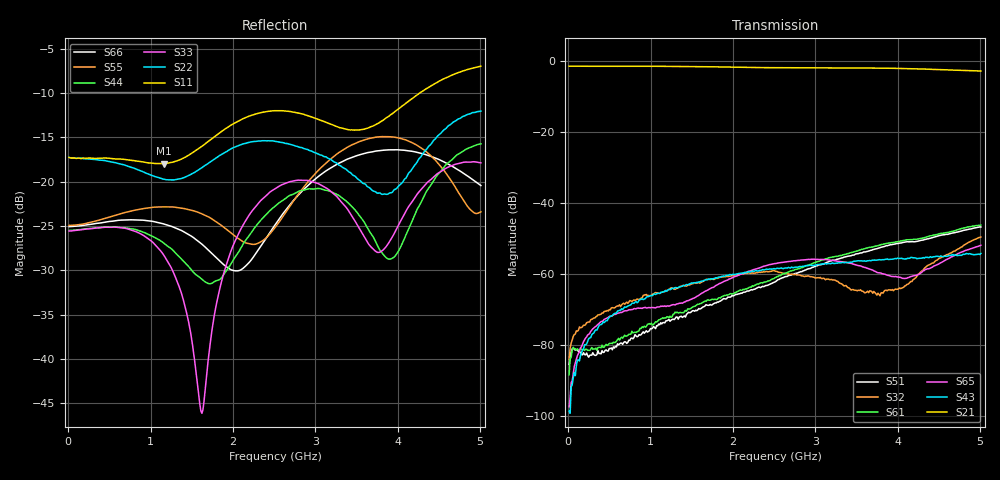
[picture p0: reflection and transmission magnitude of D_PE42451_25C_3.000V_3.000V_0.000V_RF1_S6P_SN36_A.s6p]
! Device ID: PE42451
! Serial: 36
! Insertion: A
! Temp: 25C
! VDD: 3.000
! Control_Hi: 100.000
! Control_Lo: 0.000
! Logic State: RF1
! Port 1: RFC
! Port 2: RF1
! Port 3: RF2
! Port 4: RF3
! Port 5: RF4
! Port 6: RF5
! V1 = 3.00
! V2 = 0.00
! V3 = 0.00
! V4 = 0.00
! IDD: 1.334020e-05
#  Hz  S  RI  R  50
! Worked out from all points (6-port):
!   401 points, 10 MHz to 5.01 GHz, reference 50 ohm
!   strongest paths, dB at 10 MHz, 1.26 GHz, 2.51 GHz, 3.76 GHz, 5.01 GHz:
!     S21: -1.4, -1.5, -1.8, -2.0, -2.8
!     S43: -98.7, -64.0, -58.6, -56.1, -54.2
!     S65: -97.5, -68.7, -57.1, -59.7, -51.9
!     S61: -88.5, -72.1, -61.1, -52.0, -46.2
!     S32: -84.2, -64.0, -59.2, -65.5, -49.6
!     S51: -85.5, -72.9, -62.3, -52.8, -46.8
!   lowest |S11| = -18.0 dB at 1.16 GHz (marker M1), VSWR 1.29, Z = 57.3 - j11.5 ohm
!   |S11| at or under -10 dB: start of sweep to 4.268 GHz
